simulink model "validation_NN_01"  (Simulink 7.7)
settings: Solver=VariableStepDiscrete  StartTime=0.0  StopTime=100  RelTol=1e-3
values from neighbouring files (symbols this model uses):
  A = [0.9944 -0.1203 -0.4302    [process_model02.m]
  B = [1 0    [process_model02.m]
  C = [1 0 0    [process_model02.m]
  D = zeros(2,2)    [process_model02.m]
  Ts = 0.1    [process_model02.m]
  x0 = [0.01 0.02 0.03]    [process_model02.m]
libraries: neural x21, simulink x6

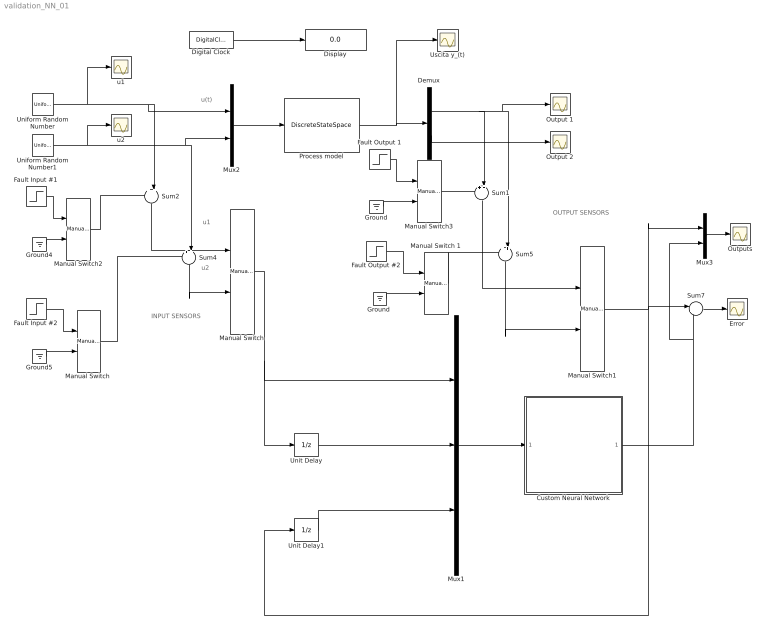
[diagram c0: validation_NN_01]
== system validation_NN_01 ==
  note: u(t)
  note: INPUT SENSORS
  note: OUTPUT SENSORS
  note: u1
  note: u2
  Custom Neural Network : Subsystem
  Demux : Demux  Outputs=2
  Digital Clock : DigitalClock  SampleTime=Ts
  Display : Display
  Error : Scope
  Fault Input #1 : Step  Time=50  After=5  SampleTime=Ts
  Fault Input #2 : Step  Time=50  After=5  SampleTime=Ts
  Fault Output #2 : Step  Time=50  After=5  SampleTime=Ts
  Fault Output 1 : Step  Time=50  After=100  SampleTime=Ts
  Ground : Ground
  "Ground " : Ground
  Ground4 : Ground
  Ground5 : Ground
  Manual Switch : simulink/Signal Routing/Manual Switch  SystemSampleTime=-1  sw=1  action=0  varsize=off
  "Manual Switch " : simulink/Signal Routing/Manual Switch  SystemSampleTime=-1  sw=0  action=0  varsize=off
  Manual Switch 1 : simulink/Signal Routing/Manual Switch  SystemSampleTime=-1  sw=0  action=0  varsize=off
  Manual Switch1 : simulink/Signal Routing/Manual Switch  SystemSampleTime=-1  sw=1  action=0  varsize=off
  Manual Switch2 : simulink/Signal Routing/Manual Switch  SystemSampleTime=-1  sw=0  action=0  varsize=off
  Manual Switch3 : simulink/Signal Routing/Manual Switch  SystemSampleTime=-1  sw=0  action=0  varsize=off
  Mux1 : Mux  Inputs=3
  Mux2 : Mux  Inputs=2
  Mux3 : Mux  Inputs=2
  Output 1 : Scope
  Output 2 : Scope
  Outputs : Scope
  Process model : DiscreteStateSpace  A=A  B=B  C=C  D=D  X0=x0  SampleTime=Ts
  Sum{1..2,4..5} (4 alike) : Sum  Inputs=++|
  Sum7 : Sum  Inputs=|+-
  Uniform Random Number : UniformRandomNumber  Seed=11  SampleTime=Ts
  Uniform Random Number1 : UniformRandomNumber  Minimum=-0.5  Maximum=0.5  Seed=13  SampleTime=Ts
  Unit Delay : UnitDelay  SampleTime=Ts
  Unit Delay1 : UnitDelay  SampleTime=Ts
  Uscita y_(t) : Scope
  u1 : Scope
  u2 : Scope
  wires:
  Digital Clock/1 -> Display/1
  Mux2/1 -> Process model/1
  Uniform Random Number/1 -> u1/1, Mux2/1, Sum2/2
  Process model/1 -> Uscita y_(t)/1, Demux/1
  Uniform Random Number1/1 -> u2/1, Mux2/2, Sum4/2
  Demux/1 -> Output 1/1, Sum5/2, Sum1/2
  Demux/2 -> Output 2/1
  Sum2/1 -> Manual Switch/1
  Sum4/1 -> Manual Switch/2
  Manual Switch/1 -> Unit Delay/1, Mux1/1
  Sum1/1 -> Manual Switch1/1
  Sum5/1 -> Manual Switch1/2
  Unit Delay1/1 -> Mux1/3
  Manual Switch1/1 -> Sum7/1, Mux3/1, Unit Delay1/1
  Mux1/1 -> Custom Neural Network/1(Input)
  Unit Delay/1 -> Mux1/2
  Custom Neural Network/1(Output) -> Sum7/2, Mux3/2
  Mux3/1 -> Outputs/1
  Sum7/1 -> Error/1
  Ground4/1 -> Manual Switch2/2
  Fault Input #1/1 -> Manual Switch2/1
  Fault Input #2/1 -> "Manual Switch "/1
  "Manual Switch "/1 -> Sum4/1
  Manual Switch2/1 -> Sum2/1
  Ground5/1 -> "Manual Switch "/2
  Ground/1 -> Manual Switch3/2
  Fault Output 1/1 -> Manual Switch3/1
  "Ground "/1 -> Manual Switch 1/2
  Fault Output #2/1 -> Manual Switch 1/1
  Manual Switch3/1 -> Sum1/1
  Manual Switch 1/1 -> Sum5/1

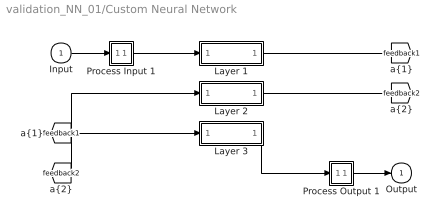
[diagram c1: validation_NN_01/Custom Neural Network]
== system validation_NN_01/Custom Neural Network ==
  Input : Inport  PortDimensions=3
  Layer 1 : Subsystem
  Layer 2 : Subsystem
  Layer 3 : Subsystem
  Process Input 1 : Subsystem
  Process Output 1 : Subsystem
  Output : Outport  InitialOutput=0
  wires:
  Input/1 -> Process Input 1/1(x)
  Process Output 1/1(y) -> Output/1
  Process Input 1/1(p) -> Layer 1/1("p{1}")
  Layer 1/1("a{1}") -> [feedback1]
  [feedback1] -> Layer 2/1("a{1} ")
  Layer 2/1("a{2}") -> [feedback2]
  [feedback2] -> Layer 3/1("a{2} ")
  Layer 3/1("a{3}") -> Process Output 1/1(a)

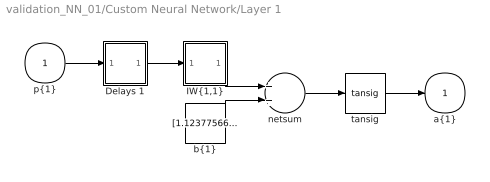
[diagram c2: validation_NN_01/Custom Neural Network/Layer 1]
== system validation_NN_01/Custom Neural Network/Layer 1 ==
  "p{1}" : Inport  PortDimensions=3
  Delays 1 : Subsystem
  "IW{1,1}" : Subsystem
  "b{1}" : Constant  Value=[1.1237756645610004;-0.054268478786377701;0.57594435392476406;-4.9243345146351123]
  netsum : Sum  Inputs=2
  tansig : neural/Transfer Functions/tansig  SystemSampleTime=-1
  "a{1}" : Outport  InitialOutput=[0;0;0;0]
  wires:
  "p{1}"/1 -> Delays 1/1("p{1}")
  Delays 1/1("pd{1,1}") -> "IW{1,1}"/1("pd{1,1}")
  "IW{1,1}"/1("iz{1,1}") -> netsum/1
  "b{1}"/1 -> netsum/2
  netsum/1 -> tansig/1
  tansig/1 -> "a{1}"/1

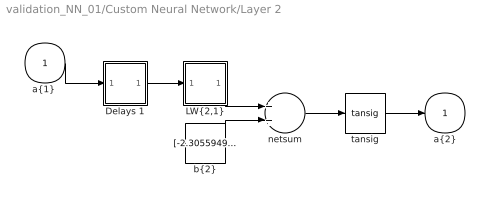
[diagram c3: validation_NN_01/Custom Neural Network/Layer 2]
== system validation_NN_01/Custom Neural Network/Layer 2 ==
  "a{1} " : Inport  PortDimensions=4
  Delays 1 : Subsystem
  "LW{2,1}" : Subsystem
  "b{2}" : Constant  Value=[-2.3055949047534914;1.3626713665317851;-0.57101867962285524;-0.099522800148013749;0.10095848160068989;0.78207591524951925;1.4007959538680181;-2.7548057782261623]
  netsum : Sum  Inputs=2
  tansig : neural/Transfer Functions/tansig  SystemSampleTime=-1
  "a{2}" : Outport  InitialOutput=[0;0;0;0;0;0;0;0]
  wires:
  "a{1} "/1 -> Delays 1/1("p{2}")
  Delays 1/1("pd{2,1}") -> "LW{2,1}"/1("ad{2,1}")
  "LW{2,1}"/1("lz{2,1}") -> netsum/1
  "b{2}"/1 -> netsum/2
  netsum/1 -> tansig/1
  tansig/1 -> "a{2}"/1

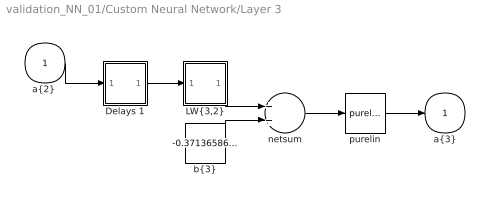
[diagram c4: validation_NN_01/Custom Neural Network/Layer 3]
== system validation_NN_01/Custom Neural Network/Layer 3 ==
  "a{2} " : Inport  PortDimensions=8
  Delays 1 : Subsystem
  "LW{3,2}" : Subsystem
  "b{3}" : Constant  Value=-0.37136586824033857
  netsum : Sum  Inputs=2
  purelin : neural/Transfer Functions/purelin  SystemSampleTime=-1
  "a{3}" : Outport  InitialOutput=0
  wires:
  "a{2} "/1 -> Delays 1/1("p{3}")
  Delays 1/1("pd{3,2}") -> "LW{3,2}"/1("ad{3,2}")
  "LW{3,2}"/1("lz{3,2}") -> netsum/1
  "b{3}"/1 -> netsum/2
  netsum/1 -> purelin/1
  purelin/1 -> "a{3}"/1

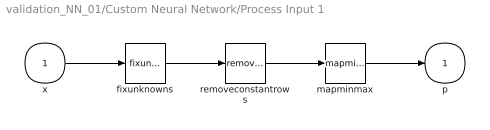
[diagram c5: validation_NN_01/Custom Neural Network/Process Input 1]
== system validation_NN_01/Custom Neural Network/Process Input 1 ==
  x : Inport  PortDimensions=3
  fixunknowns : neural/Processing Functions/fixunknowns  SystemSampleTime=-1  inputSize=3  indices=[1 2 3]
  mapminmax : neural/Processing Functions/mapminmax  SystemSampleTime=-1  xmin=[-1.137661454327592;-1.1106929140419901;-31.095443858794159]  xmax=[1.1540492640826692;1.122893357889289;32.607744268199028]  ymin=-1  ymax=1
  removeconstantrows : neural/Processing Functions/removeconstantrows  SystemSampleTime=-1  inputSize=3  keep=[1 2 3]
  p : Outport  PortDimensions=3
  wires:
  x/1 -> fixunknowns/1
  fixunknowns/1 -> removeconstantrows/1
  removeconstantrows/1 -> mapminmax/1
  mapminmax/1 -> p/1

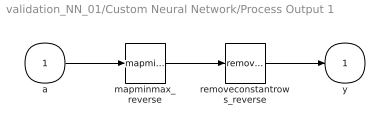
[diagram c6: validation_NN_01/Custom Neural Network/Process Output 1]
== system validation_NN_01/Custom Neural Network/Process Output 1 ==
  a : Inport  PortDimensions=1
  mapminmax_reverse : neural/Processing Functions/mapminmax_reverse  SystemSampleTime=-1  xmin=-31.173256733227603  xmax=32.664397268400201  ymin=-1  ymax=1
  removeconstantrows_reverse : neural/Processing Functions/removeconstantrows_reverse  SystemSampleTime=-1  inputSize=1  constants=zeros(0,1)  rearrange=1
  y : Outport  PortDimensions=1
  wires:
  a/1 -> mapminmax_reverse/1
  mapminmax_reverse/1 -> removeconstantrows_reverse/1
  removeconstantrows_reverse/1 -> y/1

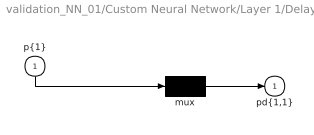
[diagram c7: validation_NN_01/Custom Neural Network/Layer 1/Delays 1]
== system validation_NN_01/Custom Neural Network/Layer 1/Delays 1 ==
  "p{1}" : Inport  PortDimensions=3
  mux : Mux  Inputs=1
  "pd{1,1}" : Outport
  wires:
  "p{1}"/1 -> mux/1
  mux/1 -> "pd{1,1}"/1

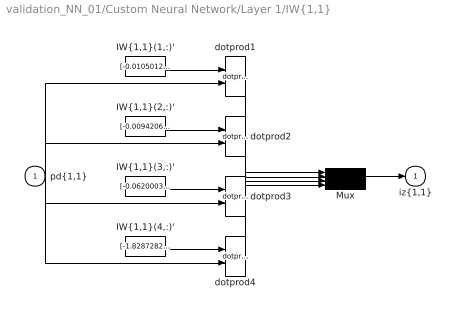
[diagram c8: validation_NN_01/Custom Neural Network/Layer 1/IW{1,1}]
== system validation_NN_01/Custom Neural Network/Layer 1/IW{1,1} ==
  "pd{1,1}" : Inport  PortDimensions=3
  "IW{1,1}(1,:)'" : Constant  Value=[-0.010501210346663943;-0.046350232521015777;-0.66458406919607949]
  "IW{1,1}(2,:)'" : Constant  Value=[-0.0094206522705928518;-0.034064818087183021;-0.57426612474193373]
  "IW{1,1}(3,:)'" : Constant  Value=[-0.062000398502087127;-0.097457836770019041;1.0232456465693076]
  "IW{1,1}(4,:)'" : Constant  Value=[-1.8287282120108412;-2.2973742278520111;3.1455267998071204]
  Mux : Mux
  dotprod{1..4} (4 alike) : neural/Weight Functions/dotprod  SystemSampleTime=-1
  "iz{1,1}" : Outport
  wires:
  "IW{1,1}(1,:)'"/1 -> dotprod1/1
  "pd{1,1}"/1 -> dotprod1/2, dotprod2/2, dotprod3/2, dotprod4/2
  dotprod1/1 -> Mux/1
  "IW{1,1}(2,:)'"/1 -> dotprod2/1
  dotprod2/1 -> Mux/2
  "IW{1,1}(3,:)'"/1 -> dotprod3/1
  dotprod3/1 -> Mux/3
  "IW{1,1}(4,:)'"/1 -> dotprod4/1
  dotprod4/1 -> Mux/4
  Mux/1 -> "iz{1,1}"/1

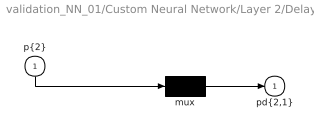
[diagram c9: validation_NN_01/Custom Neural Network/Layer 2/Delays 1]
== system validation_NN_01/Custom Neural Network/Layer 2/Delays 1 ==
  "p{2}" : Inport  PortDimensions=4
  mux : Mux  Inputs=1
  "pd{2,1}" : Outport
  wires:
  "p{2}"/1 -> mux/1
  mux/1 -> "pd{2,1}"/1

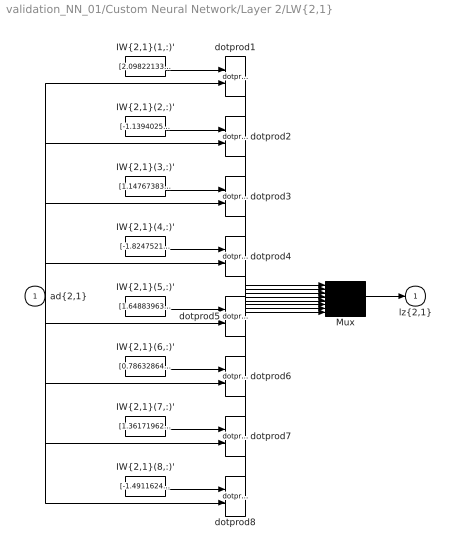
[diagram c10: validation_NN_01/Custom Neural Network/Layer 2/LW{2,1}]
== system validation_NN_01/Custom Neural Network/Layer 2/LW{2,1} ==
  "ad{2,1}" : Inport  PortDimensions=4
  "IW{2,1}(1,:)'" : Constant  Value=[2.098221331077557;0.45092990943683631;-0.052082272447184205;-0.038350945484869184]
  "IW{2,1}(2,:)'" : Constant  Value=[-1.1394025863919079;-2.1528928737433151;-0.29289688288123317;0.2695037801284455]
  "IW{2,1}(3,:)'" : Constant  Value=[1.1476738353196907;0.27086268761525978;1.4651162060837031;-0.85246368108332449]
  "IW{2,1}(4,:)'" : Constant  Value=[-1.8247521425685163;-0.60377890384517463;0.49401643562939951;1.1838578745068769]
  "IW{2,1}(5,:)'" : Constant  Value=[1.6488396331037367;-1.4644286410496272;0.79416418623969387;-0.32884994903976533]
  "IW{2,1}(6,:)'" : Constant  Value=[0.78632864001132419;-0.75329693273970155;-2.3404763728688596;1.243867874989699]
  "IW{2,1}(7,:)'" : Constant  Value=[1.3617196286206696;0.20997547932744495;-1.4297139156985137;-0.060007617806143151]
  "IW{2,1}(8,:)'" : Constant  Value=[-1.4911624483363064;-1.3342490977462667;-1.2238317148487317;-0.3970708722795096]
  Mux : Mux  Inputs=8
  dotprod{1..8} (8 alike) : neural/Weight Functions/dotprod  SystemSampleTime=-1
  "lz{2,1}" : Outport
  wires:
  "IW{2,1}(1,:)'"/1 -> dotprod1/1
  "ad{2,1}"/1 -> dotprod1/2, dotprod2/2, dotprod3/2, dotprod4/2, dotprod5/2, dotprod6/2, dotprod7/2, dotprod8/2
  dotprod1/1 -> Mux/1
  "IW{2,1}(2,:)'"/1 -> dotprod2/1
  dotprod2/1 -> Mux/2
  "IW{2,1}(3,:)'"/1 -> dotprod3/1
  dotprod3/1 -> Mux/3
  "IW{2,1}(4,:)'"/1 -> dotprod4/1
  dotprod4/1 -> Mux/4
  "IW{2,1}(5,:)'"/1 -> dotprod5/1
  dotprod5/1 -> Mux/5
  "IW{2,1}(6,:)'"/1 -> dotprod6/1
  dotprod6/1 -> Mux/6
  "IW{2,1}(7,:)'"/1 -> dotprod7/1
  dotprod7/1 -> Mux/7
  "IW{2,1}(8,:)'"/1 -> dotprod8/1
  dotprod8/1 -> Mux/8
  Mux/1 -> "lz{2,1}"/1

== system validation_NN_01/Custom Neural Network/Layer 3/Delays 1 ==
  "p{3}" : Inport  PortDimensions=8
  mux : Mux  Inputs=1
  "pd{3,2}" : Outport
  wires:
  "p{3}"/1 -> mux/1
  mux/1 -> "pd{3,2}"/1

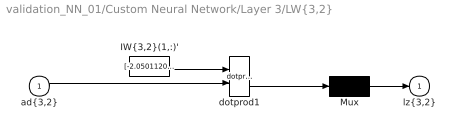
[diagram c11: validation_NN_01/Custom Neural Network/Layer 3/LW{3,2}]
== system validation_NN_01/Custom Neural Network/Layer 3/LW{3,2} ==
  "ad{3,2}" : Inport  PortDimensions=8
  "IW{3,2}(1,:)'" : Constant  Value=[-2.0501120171286527;-0.22065951383706567;-0.10718725516314385;-0.073412956754603506;0.52739347149779214;0.0092960585497072687;-0.96476250364435068;0.29489839798372447]
  Mux : Mux  Inputs=1
  dotprod1 : neural/Weight Functions/dotprod  SystemSampleTime=-1
  "lz{3,2}" : Outport
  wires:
  "IW{3,2}(1,:)'"/1 -> dotprod1/1
  "ad{3,2}"/1 -> dotprod1/2
  dotprod1/1 -> Mux/1
  Mux/1 -> "lz{3,2}"/1
